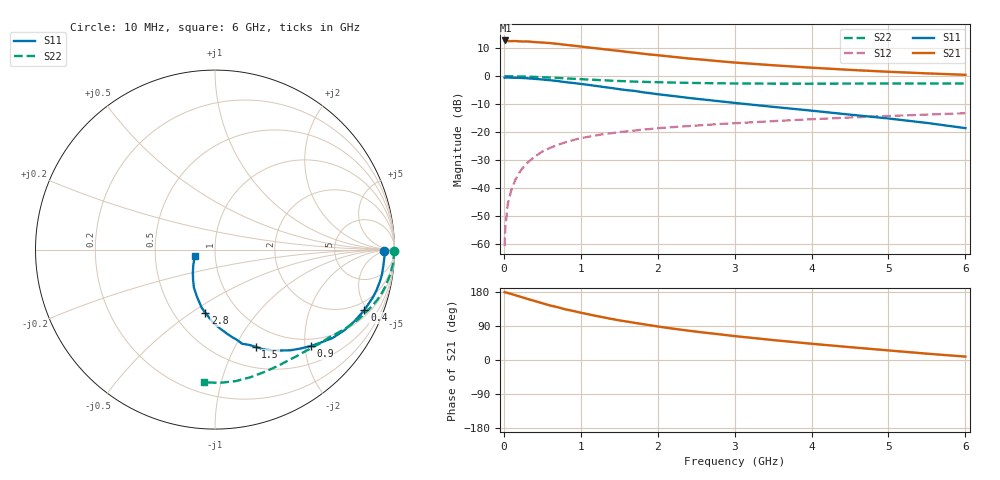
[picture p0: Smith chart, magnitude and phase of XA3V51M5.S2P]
! SIEMENS Discrete & RF Semiconductors
! BFY180
! Si NPN RF Bipolar Junction Transistor in MICRO-X
! VCE = 3.5 V  IC = 1.5 mA
! Common Emitter S-Parameters:  May  1997
# GHz  S  MA  R  50
!  f  S11  S21  S12  S22
! GHz  MAG  ANG  MAG  ANG  MAG  ANG  MAG  ANG
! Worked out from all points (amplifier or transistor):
!   36 points, 10 MHz to 6 GHz, reference 50 ohm
!   highest |S21| = 12.8 dB at 20 MHz (marker M1)
!   |S21| within 3 dB of that: start of sweep to 1.257 GHz
!   unconditionally stable (mu >= 1): 3.235 GHz to end of sweep
!   at 250 MHz: K = 0.10, MSG = 22.6 dB, |S12| = -32.7 dB
!   at 1.4 GHz: K = 0.60, MSG = 14.9 dB, |S12| = -20.4 dB
!   at 6 GHz: K = 1.07, MAG = 5.3 dB, |S12| = -13.3 dB
!   S11 on the Smith chart (normalised r, x): 10 MHz: 33, -5; 400 MHz: 1.37, -4.77; 900 MHz: 0.84, -2.12; 1.5 GHz: 0.74, -1.21; 2.8 GHz: 0.71, -0.57; 6 GHz: 0.80, -0.06
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0.01  0.9425 -0.5  4.255 179.2  0.0009 92.4  0.9954 -0.3
0.02  0.9479 -1.1  4.378 178.4  0.002 91.0  0.9994 -0.6
0.05  0.9445 -2.7  4.263 177.0  0.005 85.0  0.9976 -1.5
0.1  0.9424 -5.5  4.259 174.1  0.0094 89.0  0.9961 -3.1
0.15  0.9404 -8.5  4.277 170.9  0.0139 84.9  0.9945 -4.6
0.3  0.9196 -16.7  4.204 161.6  0.0276 79.6  0.9823 -9.0
0.4  0.8981 -22.0  4.097 155.8  0.0362 75.6  0.9732 -11.8
0.6  0.849 -32.0  3.931 143.9  0.0519 69.2  0.9469 -17.1
0.8  0.7848 -41.3  3.659 133.7  0.0654 63.2  0.9153 -21.8
0.9  0.7568 -45.3  3.538 129.5  0.0717 60.6  0.9008 -24.0
1.1  0.7007 -53.2  3.279 120.6  0.0822 56.1  0.8718 -27.9
1.2  0.6696 -57.1  3.17 116.3  0.0871 54.1  0.8592 -29.8
1.5  0.5868 -67.3  2.844 104.6  0.0996 49.3  0.8215 -34.8
1.8  0.5178 -76.3  2.541 94.9  0.1104 45.7  0.7954 -39.2
2  0.4761 -81.5  2.383 88.4  0.117 43.2  0.7828 -42.1
2.2  0.4425 -86.1  2.229 82.7  0.1226 41.2  0.7702 -44.8
2.6  0.3818 -94.7  1.973 72.4  0.1332 37.9  0.7529 -50.0
2.8  0.3562 -98.8  1.858 67.9  0.1392 36.3  0.7483 -52.5
3.5  0.2826 -110.7  1.573 52.6  0.1566 31.2  0.7369 -61.2
4.5  0.205 -126.7  1.3 33.9  0.1821 24.0  0.7379 -74.1
5.5  0.1455 -145.9  1.125 16.7  0.2056 16.5  0.7428 -87.9
6  0.1175 -161.6  1.06 9.0  0.2169 12.3  0.7421 -94.9
